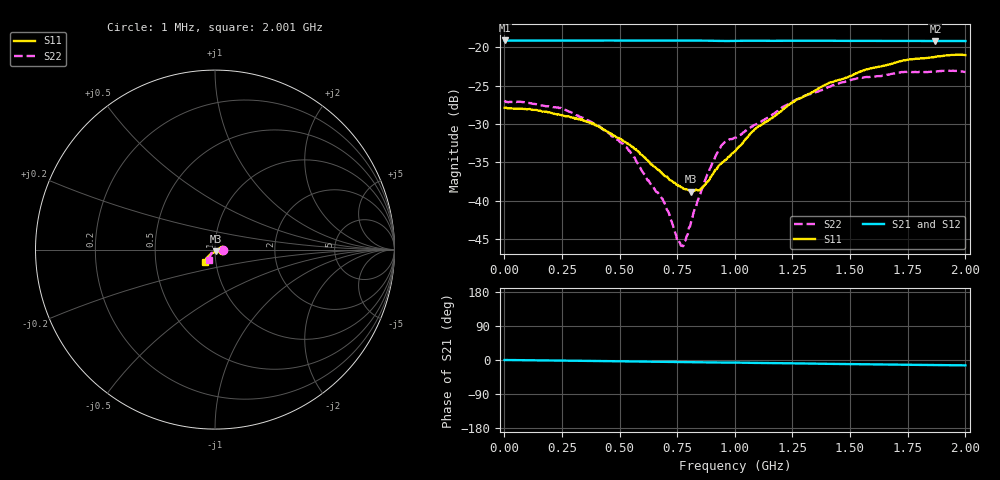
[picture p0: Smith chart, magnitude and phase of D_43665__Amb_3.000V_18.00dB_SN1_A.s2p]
! device id: 43665_
! dir: \\malibu\benchdata\1_engineers\tn_data\43665_75ohm\new\sparar\43665_\amb\3p000v\18p00db
! Serial: 1
! Insertion: A
! Temp: Amb
! VDD: 3.000V
! Attenuation Step: 18.00dB
! IDD: 1.445634e+00mA
! FILE NAME
! DATE 03-27-2009 08:37:45
! CORRECTED  DATA
#  Hz  S  RI  R  75
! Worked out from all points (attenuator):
!   401 points, 1 MHz to 2.001 GHz, reference 75 ohm
!   highest |S21| = -19.13 dB at 1 MHz (marker M1); lowest = -19.2 dB at 1.871 GHz (marker M2)
!   lowest |S11| = -38.8 dB at 811 MHz (marker M3), VSWR 1.02, Z = 75.7 - j1.6 ohm
!   |S11| at or under -10 dB: start of sweep to end of sweep
!   |S22| runs from -45.9 to -23.1 dB; largest |S21 - S12| = 0.00048
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1000000  0.0404 -0.000427  0.1106 -5.51e-05  0.1106 -3.32e-05  0.045 -0.000458
2.36e8  0.0365 -0.000551  0.1104 -0.00288  0.1104 -0.00287  0.0398 0.00565
3.36e8  0.0339 -0.00143  0.1103 -0.00418  0.1104 -0.00409  0.0341 0.00706
4.06e8  0.0306 -0.00145  0.1103 -0.00503  0.1103 -0.00495  0.03 0.00687
5.21e8  0.024 -0.00329  0.1102 -0.0067  0.1103 -0.00658  0.0226 0.00457
6.71e8  0.0144 -0.00664  0.1101 -0.00864  0.1101 -0.00851  0.011 0.000187
7.06e8  0.0121 -0.00773  0.11 -0.00915  0.1101 -0.009  0.00867 -0.000874
7.61e8  0.00835 -0.00931  0.11 -0.01  0.11 -0.00984  0.00405 -0.00353
7.81e8  0.00694 -0.00972  0.1099 -0.0104  0.11 -0.0102  0.0021 -0.00497
8.11e8  0.00453 -0.0105  0.1099 -0.0109  0.1099 -0.0106  -9.73e-05 -0.00735
8.56e8  0.00103 -0.0121  0.1097 -0.0116  0.1098 -0.0113  -0.00332 -0.0113
9.26e8  -0.00515 -0.0157  0.1091 -0.0127  0.1092 -0.0124  -0.0109 -0.0177
9.51e8  -0.00674 -0.0166  0.109 -0.0128  0.1091 -0.0125  -0.0149 -0.0184
1.001e9  -0.0106 -0.0181  0.1091 -0.0131  0.1092 -0.0128  -0.019 -0.0175
1.096e9  -0.0193 -0.0231  0.1091 -0.0148  0.1093 -0.0144  -0.0211 -0.0237
1.246e9  -0.0302 -0.0311  0.1088 -0.0168  0.109 -0.0165  -0.0265 -0.035
1.336e9  -0.0357 -0.0363  0.1087 -0.0181  0.109 -0.0178  -0.0292 -0.0407
1.406e9  -0.0407 -0.0416  0.1084 -0.0194  0.1088 -0.0192  -0.0292 -0.0468
1.521e9  -0.0469 -0.0479  0.1079 -0.0208  0.1083 -0.0206  -0.0337 -0.0521
1.671e9  -0.0528 -0.0567  0.1074 -0.0228  0.1077 -0.0228  -0.0343 -0.057
1.871e9  -0.0561 -0.0658  0.1067 -0.0253  0.1068 -0.0252  -0.0342 -0.0606
2.001e9  -0.0559 -0.0691  0.1063 -0.0268  0.1064 -0.027  -0.033 -0.0604
